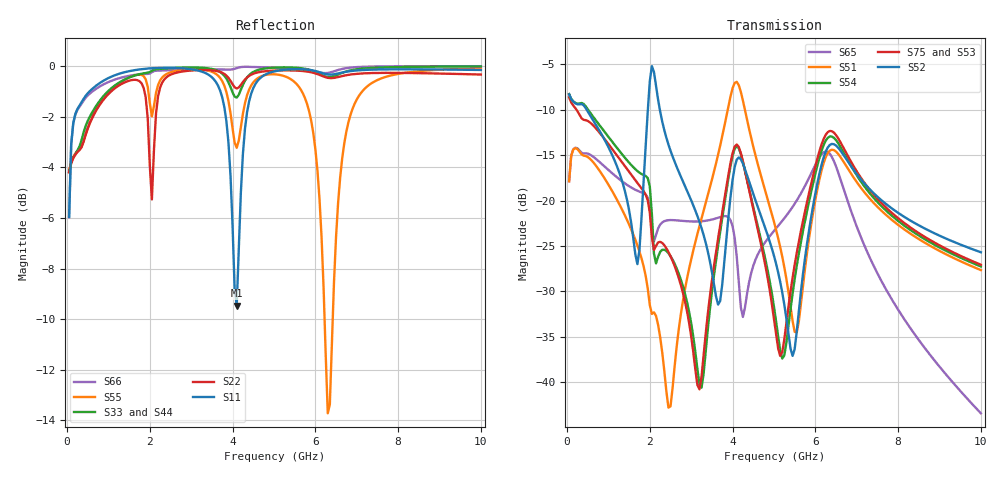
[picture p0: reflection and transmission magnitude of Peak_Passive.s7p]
! Created Fri Dec 28 23:16:22 2018
# ghz S ma R 50
! 7 Port Network Data from SP1.SP block
! freq  magS11  angS11  magS12  angS12  magS13  angS13  magS14  angS14
!  magS15  angS15  magS16  angS16  magS17  angS17
!  magS21  angS21
!  magS22  angS22  magS23  angS23  magS24  angS24  magS25  angS25
!  magS26  angS26  magS27  angS27
!  magS31  angS31  magS32  angS32
!  magS33  angS33  magS34  angS34  magS35  angS35  magS36  angS36
!  magS37  angS37
!  magS41  angS41  magS42  angS42  magS43  angS43
!  magS44  angS44  magS45  angS45  magS46  angS46  magS47  angS47
!  magS51  angS51  magS52  angS52  magS53  angS53  magS54  angS54
!  magS55  angS55  magS56  angS56  magS57  angS57
!  magS61  angS61
!  magS62  angS62  magS63  angS63  magS64  angS64  magS65  angS65
!  magS66  angS66  magS67  angS67
!  magS71  angS71  magS72  angS72
!  magS73  angS73  magS74  angS74  magS75  angS75  magS76  angS76
!  magS77  angS77
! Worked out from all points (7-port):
!   200 points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, 50 MHz to 10 GHz, reference 50 ohm
!   strongest paths, dB at 50 MHz, 2.55 GHz, 5.05 GHz, 7.55 GHz, 10 GHz:
!     S52: -8.3, -15.2, -26.9, -19.8, -25.7
!     S75: -8.6, -26.6, -34.7, -20.1, -27.1
!     S53: -8.6, -26.6, -34.7, -20.1, -27.1
!     S54: -8.3, -26.5, -33.3, -20.4, -27.3
!     S51: -17.9, -40.6, -23.2, -20.9, -27.7
!     S65: -17.9, -22.2, -23.1, -28.5, -43.4
!   lowest |S11| = -9.5 dB at 4.1 GHz (marker M1), VSWR 2.01, Z = 24.8 + j0.0889 ohm
!   |S11| at or under -10 dB: nowhere
